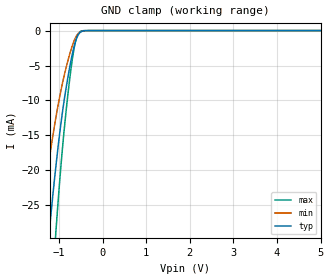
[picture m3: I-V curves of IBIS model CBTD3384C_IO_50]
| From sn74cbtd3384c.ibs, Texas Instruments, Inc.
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[Model]   CBTD3384C_IO_50
Model_type  Terminator
| variable   typ   min   max
C_comp   8.10pF   4.24pF   16.27pF
| C_tri-state   8.10pF   4.24pF   16.27pF
[Temperature Range]   40   100   -40
| Ambient temperature   25   85   -40
[Voltage range]   5   4.5   5.5
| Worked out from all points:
|   GND clamp passes 1 mA (typ) near -0.59 V on its own axis
[GND Clamp]
| CBTD3384C_IO_50
|   Voltage   I(typ)   I(min)   I(max)
-5V       -402.2mA   -300.9mA   -511.8mA
-1.455V   -45.58mA   -29.39mA   -67.35mA
-1.43V    -43.65mA   -28.12mA   -64.62mA
-1.22V    -28.62mA   -18.31mA   -42.73mA
-1.075V   -19.63mA   -12.57mA   -29.14mA
-905mV    -10.99mA   -7.102mA   -15.78mA
-825mV    -7.763mA   -5.015mA   -10.81mA
-735mV    -4.616mA   -2.962mA   -5.968mA
-680mV    -2.974mA   -1.899mA   -3.513mA
-615mV    -1.454mA   -943.6uA   -1.408mA
-495mV    -166.4uA   -140uA     -77.2uA
5V        570.7pA    1.883nA    133.1pA
